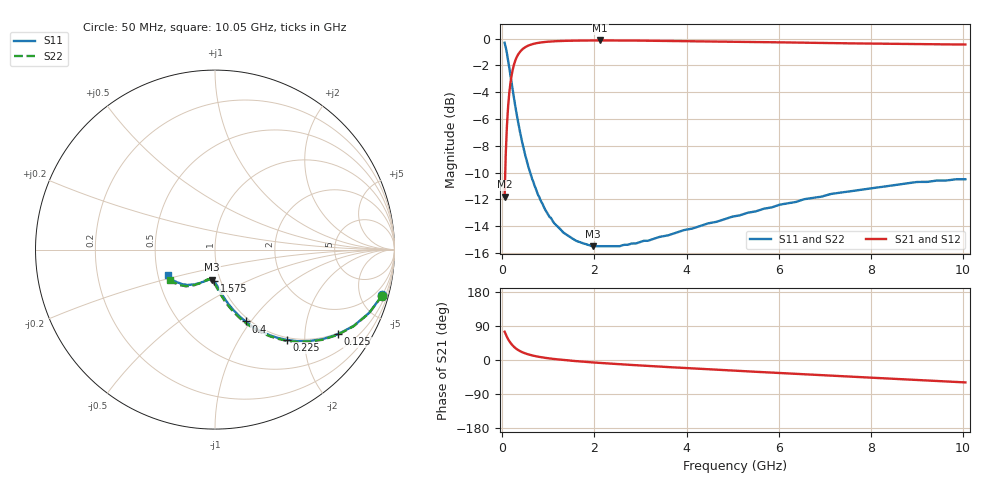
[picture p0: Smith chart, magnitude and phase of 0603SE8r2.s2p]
! AVX Thin Film Operation		Date: August 2001
! Description: Accu-P® Series, Thin Film, SMD, RF Capacitor
! Part Number: 06035J8R2BBT
! 50 MHz  -  10.05 GHz
! Serial Measurements
# mhz S db R 50
!	S11		S21		S12		S22
!	dB	Phase	dB	Phase	dB	Phase	dB	Phase
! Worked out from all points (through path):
!   401 points, 50 MHz to 10.05 GHz, reference 50 ohm
!   highest |S21| = -0.13 dB at 2.125 GHz (marker M1); lowest = -11.8 dB at 50 MHz (marker M2)
!   group delay of S21, straight-line fit = 21.5 ps
!   lowest |S11| = -15.5 dB at 1.975 GHz (marker M3), VSWR 1.40, Z = 45.9 - j15.8 ohm
!   |S11| at or under -10 dB: 605.1 MHz to end of sweep
!   |S22| runs from -15.5 to -0.3 dB; largest |S21 - S12| = 0
!   S11 on the Smith chart (normalised r, x): 50 MHz: 0.96, -7.32; 125 MHz: 0.96, -2.93; 225 MHz: 0.96, -1.65; 400 MHz: 0.96, -0.94; 1.575 GHz: 0.93, -0.34; 10.05 GHz: 0.56, -0.18
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50  -0.30 -15.3  -11.80 74.6  -11.80 74.6  -0.30 -15.4
75  -0.65 -22.3  -8.59 67.6  -8.59 67.6  -0.65 -22.5
125  -1.60 -34.6  -5.12 55.2  -5.12 55.2  -1.60 -34.9
175  -2.70 -44.1  -3.35 45.7  -3.35 45.7  -2.70 -44.5
225  -3.82 -51.4  -2.33 38.2  -2.33 38.2  -3.82 -52.0
300  -5.41 -59.6  -1.48 30.0  -1.48 30.0  -5.41 -60.3
400  -7.23 -67.0  -0.92 22.5  -0.92 22.5  -7.23 -67.9
500  -8.74 -72.0  -0.63 17.3  -0.63 17.3  -8.74 -73.2
600  -9.94 -75.6  -0.47 13.6  -0.47 13.6  -9.94 -77.0
750  -11.43 -79.7  -0.33 9.4  -0.33 9.4  -11.43 -81.3
900  -12.54 -82.7  -0.25 6.2  -0.25 6.2  -12.54 -84.5
1175  -13.95 -86.9  -0.18 1.9  -0.18 1.9  -13.95 -89.0
1575  -15.04 -91.4  -0.14 -2.7  -0.14 -2.7  -15.04 -93.5
1725  -15.25 -92.9  -0.14 -4.2  -0.14 -4.2  -15.25 -95.1
1975  -15.50 -95.2  -0.13 -6.5  -0.13 -6.5  -15.50 -97.3
2125  -15.50 -96.5  -0.13 -7.8  -0.13 -7.8  -15.50 -98.4
2550  -15.50 -100.0  -0.13 -11.2  -0.13 -11.2  -15.50 -102.0
3400  -14.82 -106.8  -0.15 -17.3  -0.15 -17.3  -14.82 -106.9
5050  -13.26 -118.4  -0.22 -28.2  -0.22 -28.2  -13.26 -117.4
6725  -11.90 -130.0  -0.31 -38.7  -0.31 -38.7  -11.89 -127.0
8400  -10.99 -141.1  -0.38 -49.1  -0.38 -49.1  -10.90 -137.1
10050  -10.50 -151.6  -0.43 -59.1  -0.43 -59.1  -10.42 -145.8
